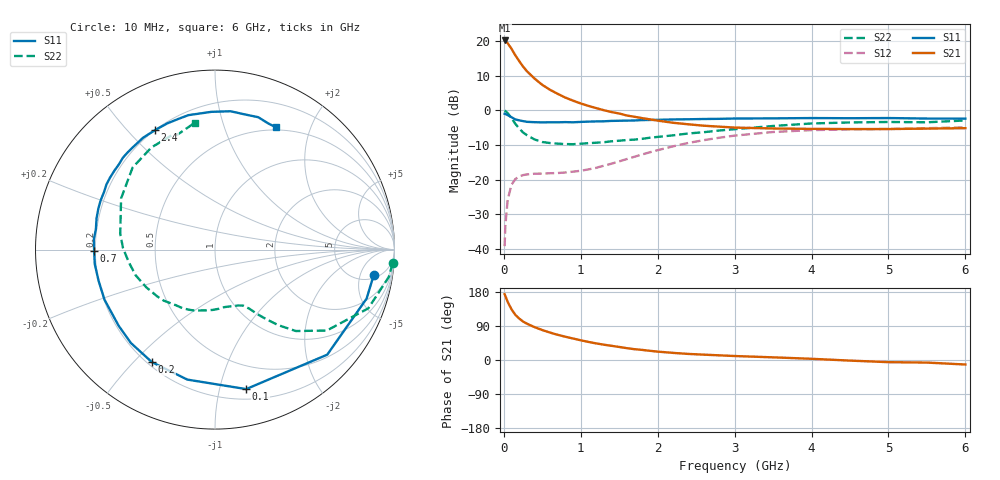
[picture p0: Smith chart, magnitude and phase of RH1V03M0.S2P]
! SIEMENS Small Signal Semiconductors
! BFR106
! Si NPN RF Bipolar Junction Transistor in SOT23
! VCE = 1 V  IC = 3 mA
! Common Emitter S-Parameters:  August  1996
# GHz  S  MA  R  50
!  f  S11  S21  S12  S22
! GHz  MAG  ANG  MAG  ANG  MAG  ANG  MAG  ANG
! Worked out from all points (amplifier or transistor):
!   36 points, 10 MHz to 6 GHz, reference 50 ohm
!   highest |S21| = 20.2 dB at 10 MHz (marker M1)
!   |S21| within 3 dB of that: start of sweep to 115.1 MHz
!   unconditionally stable (mu >= 1): 686.7 MHz to end of sweep
!   at 250 MHz: K = 0.40, MSG = 15.7 dB, |S12| = -18.7 dB
!   at 1.4 GHz: K = 1.27, MAG = 4.4 dB, |S12| = -15.4 dB
!   at 6 GHz: K = 1.03, MAG = -1.1 dB, |S12| = -4.9 dB
!   S11 on the Smith chart (normalised r, x): 10 MHz: 6, -8; 100 MHz: 0.28, -1.21; 200 MHz: 0.22, -0.56; 700 MHz: 0.20, -0.00; 2.4 GHz: 0.20, +0.60; 6 GHz: 0.47, +1.51
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0.01  0.8956 -9.1  10.27 173.8  0.0109 86.2  0.9919 -4.4
0.02  0.8877 -17.9  10.18 169.0  0.0219 81.4  0.9809 -8.9
0.05  0.8566 -43.1  9.377 153.2  0.0512 66.9  0.9143 -21.0
0.1  0.7963 -77.4  7.768 133.8  0.0844 51.1  0.7691 -35.9
0.15  0.7405 -102.0  6.244 119.0  0.1019 39.8  0.6394 -45.2
0.2  0.7188 -119.3  5.163 109.4  0.1109 33.8  0.5482 -50.1
0.25  0.7003 -132.0  4.306 101.5  0.1161 29.5  0.4799 -53.7
0.3  0.6842 -141.7  3.69 95.9  0.1188 27.3  0.4383 -56.2
0.4  0.676 -155.6  2.883 86.7  0.1216 25.1  0.3801 -59.9
0.5  0.6715 -165.1  2.341 79.0  0.1221 24.9  0.3495 -63.3
0.6  0.6747 -173.1  1.989 72.4  0.1236 26.0  0.3375 -67.2
0.7  0.6735 -179.5  1.737 66.5  0.1244 28.3  0.3311 -71.7
0.9  0.6734 170.2  1.384 56.7  0.1303 34.1  0.3248 -81.2
1.1  0.6888 160.7  1.162 47.7  0.1404 40.7  0.3361 -91.9
1.6  0.7124 141.9  0.844 31.2  0.1983 51.5  0.3734 -119.0
2.2  0.7409 122.8  0.663 18.8  0.3028 49.4  0.4364 -151.1
2.4  0.745 116.6  0.63 16.0  0.339 46.6  0.4642 -161.9
3  0.7636 101.2  0.565 10.5  0.4324 35.2  0.5353 170.6
3.5  0.7678 91.5  0.548 7.0  0.4877 25.3  0.5959 151.4
4.5  0.7713 77.3  0.538 -1.6  0.5324 7.8  0.6703 121.9
5.5  0.7629 67.1  0.546 -6.8  0.5542 -2.1  0.6739 108.0
6  0.7614 63.5  0.554 -11.9  0.5686 -8.9  0.7161 99.0
